| IBIS file stm32h563_573_ufbga169-smps.ibs
[IBIS ver] 4.2
[File name] stm32h563_573_ufbga169-smps.ibs
[File Rev] 1.1
[Date] 07-05-2024
[Source] Data Created at STMicroelectronics
[Notes]  File originated from ELDO simulations.
[Disclaimer]  This information is for modeling purpose only and is
   not guaranteed. The information is subject to change without
   notice.
[Copyright] Copyright 2024 STMicroelectronics Inc.
|   Component stm32h563_573_ufbga169-smps
[Component] stm32h563_573_ufbga169-smps
[Manufacturer] STMicroelectronics
[Package]
| variable   typ   min   max
R_pkg  0  NA  NA
L_pkg  0  NA  NA
C_pkg  0  NA  NA
[Pin]   signal_name   model_name
A1  PI7  io8_ft_i3c_spi
A2  PI6  io8_ft_i3c_spi
A3  VDD  power
A4  VCAP  nc
A5  PB4  io8_ft_i3c_spi
A6  VDDIO2  power
A7  PD5  io8_ft_i3c_spi
A8  VDD  power
A9  PC11  io8_ft_i3c_spi
A10  PC10  io8_ft_i3c_spi
A11  VDD  power
A12  PI3  io8_ft_i3c_spi
A13  PH15  io8_ft_i3c_spi
B1  VDD  power
B2  VSS  gnd
B3  PI5  io8_ft_i3c_spi
B4  VSS  gnd
B5  BOOT0  vpphv
B6  PG15  io8_ft_i3c_spi
B7  PD7  io8_ft_i3c_spi
B8  VSS  gnd
B9  PD1  io8_ft_i3c_spi
B10  PA15  io8_ft_i3c_spi
B11  VSS  gnd
B12  PI0  io8_ft_i3c_spi
B13  PA12  io8usb_ft_i3c_spi_phy
C1  VBAT  power
C2  PE5  io8_ft_i3c_spi
C3  PE2  io8_ft_i3c_spi
C4  PI4  io8_ft_i3c_spi
C5  PE1  io8_ft_i3c_spi
C6  PB6  io8_ft_i3c_spi
C7  PG10  io8_ft_i3c_spi
C8  PD3  io8_ft_i3c_spi
C9  PD0  io8_ft_i3c_spi
C10  PA14  io8_ft_i3c_spi
C11  PI1  io8_ft_i3c_spi
C12  PH13  io8_ft_i3c_spi
C13  PA11  io8usb_ft_i3c_spi_phy
D1  PC14-OSC32_IN  io8_ft_i3c_spi
D2  PE6  io8_ft_i3c_spi
D3  PE4  io8_ft_i3c_spi
D4  PE3  io8_ft_i3c_spi
D5  PE0  io8_ft_i3c_spi
D6  PB7  io8_ft_i3c_spi
D7  PG12  io8_ft_i3c_spi
D8  PD4  io8_ft_i3c_spi
D9  PC12  io8_ft_i3c_spi
D10  PI2  io8_ft_i3c_spi
D11  PH14  io8_ft_i3c_spi
D12  PA13  io8_ft_i3c_spi
D13  VDD  power
E1  PC15-OSC32_OUT  io8_ft_i3c_spi
E2  PF0  io8_ft_i3c_spi
E3  PC13  io8_ft_i3c_spi
E4  PI8  io8_ft_i3c_spi
E5  PB9  io8_ft_i3c_spi
E6  PB5  io8_ft_i3c_spi
E7  PG9  io8_ft_i3c_spi
E8  PD2  io8_ft_i3c_spi
E9  PC8  io8_ft_i3c_spi
E10  PA8  io8_ft_i3c_spi
E11  PA10  io8_ft_i3c_spi
E12  VSS  gnd
E13  VDDUSB  power
F1  PF7  io8_ft_i3c_spi
F2  VSS  gnd
F3  PF1  io8_ft_i3c_spi
F4  PF2  io8_ft_i3c_spi
F5  PB8  io8_ft_i3c_spi
F6  PB3  io8_ft_i3c_spi
F7  PD6  io8_ft_i3c_spi
F8  PG5  io8_ft_i3c_spi
F9  PG7  io8_ft_i3c_spi
F10  PC6  io8_ft_i3c_spi
F11  PC7  io8_ft_i3c_spi
F12  PC9  io8_ft_i3c_spi
F13  PA9  io8_ft_i3c_spi
G1  VDD  power
G2  PF9  io8_ft_i3c_spi
G3  PF5  io8_ft_i3c_spi
G4  PF8  io8_ft_i3c_spi
G5  PF4  io8_ft_i3c_spi
G6  PF3  io8_ft_i3c_spi
G7  PF6  io8_ft_i3c_spi
G8  PD13  io8_ft_i3c_spi
G9  PG3  io8_ft_i3c_spi
G10  PD15  io8_ft_i3c_spi
G11  PG4  io8_ft_i3c_spi
G12  PG6  io8_ft_i3c_spi
G13  PG8  io8_ft_i3c_spi
H1  PH0-OSC_IN  io8_ft_i3c_spi
H2  VSS  gnd
H3  NRST  ioreset_ft_v33
H4  PF10  io8_ft_i3c_spi
H5  PA1  io8_ft_spi_tamp
H6  PB1  io8_ft_spi
H7  PF13  io8_ft_spi
H8  PD11  io8_ft_i3c_spi
H9  PD9  io8_ft_i3c_spi
H10  PB15  io8_ft_spi
H11  PD12  io8_ft_i3c_spi
H12  PD14  io8_ft_i3c_spi
H13  PG2  io8_ft_i3c_spi
J1  PH1  io8_ft_i3c_spi
J2  PC0  io8_ft_spi
J3  PC1  io8_ft_spi
J4  PH2  io8_ft_i3c_spi
J5  PA5  io8_ft_spi
J6  PF11  io8_ft_spi
J7  PF15  io8_ft_i3c_spi
J8  PE8  io8_ft_i3c_spi
J9  PE14  io8_ft_i3c_spi
|J10  PB14  io8usb_ft_pd
J10  PB14 nc
J11  PD8  io8_ft_i3c_spi
J12  VSS  gnd
J13  VDD  power
K1  PC2  io8_ft_spi
K2  PC3  io8_ft_spi
K3  PA0  io8_ft_spi
K4  PA3  io8_ft_spi
K5  PA7  io8_ft_spi
K6  PF12  io8_ft_spi
K7  PG1  io8_ft_i3c_spi
K8  PE13  io8_ft_i3c_spi
K9  PB10  io8_ft_i3c_spi
K10  PH10  io8_ft_i3c_spi
K11  PB12  io8_ft_i3c_spi
|K12  PB13  io8usb_ft_pd
K12  PB13  nc
K13  PD10  io8_ft_i3c_spi
L1  VSSA  nc
L2  VREFM  nc
L3  PA2  io8_ft_spi
L4  PH5  io8_ft_i3c_spi
L5  PC4  io8_ft_spi
L6  PF14  io8_ft_spi
L7  PE7  io8_ft_i3c_spi
L8  PE10  io8_ft_i3c_spi
L9  PE15  io8_ft_i3c_spi
L10  PB11  io8_ft_i3c_spi
L11  PH7  io8_ft_i3c_spi
L12  PH12  io8_ft_i3c_spi
L13  PH11  io8_ft_i3c_spi
M1  VDDA  nc
M2  VREFP  nc
M3  VSS  gnd
M4  PA4  io8_ft_spi
M5  PC5  io8_ft_spi
M6  PG0  io8_ft_i3c_spi
M7  VSS  gnd
M8  PE11  io8_ft_i3c_spi
M9  PE12  io8_ft_i3c_spi
M10  VSSSMPS  nc
M11  VSS  gnd
M12  PH8  io8_ft_i3c_spi
M13  PH9  io8_ft_i3c_spi
N1  PH4  io8_ft_i3c_spi
N2  PH3  io8_ft_i3c_spi
N3  VDD  power
N4  PA6  io8_ft_spi
N5  PB0  io8_ft_spi
N6  PB2  io8_ft_i3c_spi
N7  VDD  power
N8  PE9  io8_ft_i3c_spi
N9  VLXSMPS  nc
N10  VDDSMPS  nc
N11  VCAP  nc
N12  VDD  power
N13  PH6  io8_ft_i3c_spi
[Package Model]   484-ufbga-7x7-169-smps-221014
[Pin Mapping]   pulldown_ref   pullup_ref   | Comment
A1  gndio  vddiom
A2  gndio  vddiom
A3  nc  vddiom
A4  nc  nc
A5  gndio  vddiom  | Depending on IO usage
| A5  gndio  vddmmc  | Depending on IO usage
A6  nc  vddmmc
A7  gndio  vddiom
A8  nc  vddiom
A9  gndio  vddiom
A10  gndio  vddiom
A11  nc  vddiom
A12  gndio  vddiom
A13  gndio  vddiom
B1  nc  vddiom
B2  gndio  nc
B3  gndio  vddiom
B4  gndio  nc
B5  gndio  vddiom  | Depending on IO usage
| B5  gndio  vddmmc  | Depending on IO usage
B6  gndio  vddiom  | Depending on IO usage
| B6  gndio  vddmmc  | Depending on IO usage
B7  gndio  vddiom  | Depending on IO usage
| B7  gndio  vddmmc  | Depending on IO usage
B8  gndio  nc
B9  gndio  vddiom
B10  gndio  vddiom
B11  gndio  nc
B12  gndio  vddiom
B13  gndio  vddiom  | Depending on IO usage
| B13  gndio  vddusb  | Depending on IO usage
C1  nc  vsw
C2  gndio  vddiom
C3  gndio  vddiom
C4  gndio  vddiom
C5  gndio  vddiom  | Depending on IO usage
| C5  gndio  vddmmc  | Depending on IO usage
C6  gndio  vddiom  | Depending on IO usage
| C6  gndio  vddmmc  | Depending on IO usage
C7  gndio  vddiom  | Depending on IO usage
| C7  gndio  vddmmc  | Depending on IO usage
C8  gndio  vddiom
C9  gndio  vddiom
C10  gndio  vddiom
C11  gndio  vddiom
C12  gndio  vddiom
C13  gndio  vddiom  | Depending on IO usage
| C13  gndio  vddusb  | Depending on IO usage
D1  gndio  vddiom  | Depending on IO usage
| D1  gndio  vsw  | Depending on IO usage
D2  gndio  vddiom
D3  gndio  vddiom
D4  gndio  vddiom
D5  gndio  vddiom  | Depending on IO usage
| D5  gndio  vddmmc  | Depending on IO usage
D6  gndio  vddiom  | Depending on IO usage
| D6  gndio  vddmmc  | Depending on IO usage
D7  gndio  vddiom  | Depending on IO usage
| D7  gndio  vddmmc  | Depending on IO usage
D8  gndio  vddiom
D9  gndio  vddiom
D10  gndio  vddiom
D11  gndio  vddiom
D12  gndio  vddiom  | Depending on IO usage
| D12  gndio  vddusb  | Depending on IO usage
D13  nc  vddiom
E1  gndio  vddiom  | Depending on IO usage
| E1  gndio  vsw  | Depending on IO usage
E2  gndio  vddiom
E3  gndio  vddiom  | Depending on IO usage
| E3  gndio  vsw  | Depending on IO usage
E4  gndio  vddiom  | Depending on IO usage
| E4  gndio  vsw  | Depending on IO usage
E5  gndio  vddiom  | Depending on IO usage
| E5  gndio  vddmmc  | Depending on IO usage
E6  gndio  vddiom  | Depending on IO usage
| E6  gndio  vddmmc  | Depending on IO usage
E7  gndio  vddiom  | Depending on IO usage
| E7  gndio  vddmmc  | Depending on IO usage
E8  gndio  vddiom
E9  gndio  vddiom
E10  gndio  vddiom
E11  gndio  vddiom  | Depending on IO usage
| E11  gndio  vddusb  | Depending on IO usage
E12  gndio  nc
E13  nc  vddusb
F1  gndio  vddiom
F2  gndio  nc
F3  gndio  vddiom
F4  gndio  vddiom
F5  gndio  vddiom  | Depending on IO usage
| F5  gndio  vddmmc  | Depending on IO usage
F6  gndio  vddiom  | Depending on IO usage
| F6  gndio  vddmmc  | Depending on IO usage
F7  gndio  vddiom  | Depending on IO usage
| F7  gndio  vddmmc  | Depending on IO usage
F8  gndio  vddiom
F9  gndio  vddiom
F10  gndio  vddiom
F11  gndio  vddiom
F12  gndio  vddiom
F13  gndio  vddiom  | Depending on IO usage
| F13  gndio  vddusb  | Depending on IO usage
G1  nc  vddiom
G2  gndio  vddiom
G3  gndio  vddiom
G4  gndio  vddiom
G5  gndio  vddiom
G6  gndio  vddiom
G7  gndio  vddiom
G8  gndio  vddiom
G9  gndio  vddiom
G10  gndio  vddiom
G11  gndio  vddiom
G12  gndio  vddiom
G13  gndio  vddiom
H1  gndio  vddiom
H2  gndio  nc
H3  gndio  vddiom
H4  gndio  vddiom
H5  gndio  vddiom
H6  gndio  vddiom
H7  gndio  vddiom
H8  gndio  vddiom
H9  gndio  vddiom
H10  gndio  vddiom
H11  gndio  vddiom
H12  gndio  vddiom
H13  gndio  vddiom
J1  gndio  vddiom
J2  gndio  vddiom
J3  gndio  vddiom
J4  gndio  vddiom
J5  gndio  vddiom
J6  gndio  vddiom
J7  gndio  vddiom
J8  gndio  vddiom
J9  gndio  vddiom
|J10  gndio  vddiom
J10  nc nc
J11  gndio  vddiom
J12  gndio  nc
J13  nc  vddiom
K1  gndio  vddiom
K2  gndio  vddiom
K3  gndio  vddiom
K4  gndio  vddiom
K5  gndio  vddiom
K6  gndio  vddiom
K7  gndio  vddiom
K8  gndio  vddiom
K9  gndio  vddiom
K10  gndio  vddiom
K11  gndio  vddiom
|K12  gndio  vddiom
K12  nc nc
K13  gndio  vddiom
L1  nc  nc
L2  nc  nc
L3  gndio  vddiom
L4  gndio  vddiom
L5  gndio  vddiom
L6  gndio  vddiom
L7  gndio  vddiom
L8  gndio  vddiom
L9  gndio  vddiom
L10  gndio  vddiom
L11  gndio  vddiom
L12  gndio  vddiom
L13  gndio  vddiom
M1  nc  nc
M2  nc  nc
M3  gndio  nc
M4  gndio  vddiom
M5  gndio  vddiom
M6  gndio  vddiom
M7  gndio  nc
M8  gndio  vddiom
M9  gndio  vddiom
M10  nc  nc
M11  gndio  nc
M12  gndio  vddiom
M13  gndio  vddiom
N1  gndio  vddiom
N2  gndio  vddiom
N3  nc  vddiom
N4  gndio  vddiom
N5  gndio  vddiom
N6  gndio  vddiom
N7  nc  vddiom
N8  gndio  vddiom
N9  nc  nc
N10  nc  nc
N11  nc  nc
N12  nc  vddiom
N13  gndio  vddiom
[Model Selector] io8_ft_i3c_spi
io8_ft_spi_ls_1v2 "io8_ft spi low speed @ 1.2V"
io8_ft_spi_ls_1v8 "io8_ft spi low speed @ 1.8V"
io8_ft_spi_ls_3v3 "io8_ft spi low speed @ 3.3V"
io8_ft_spi_ms_1v2 "io8_ft spi med speed @ 1.2V"
io8_ft_spi_ms_1v8 "io8_ft spi med speed @ 1.8V"
io8_ft_spi_ms_3v3 "io8_ft spi med speed @ 3.3V"
io8_ft_spi_fs_1v2 "io8_ft spi fast speed @ 1.2V"
io8_ft_spi_fs_1v8 "io8_ft spi fast speed @ 1.8V"
io8_ft_spi_fs_3v3 "io8_ft spi fast speed @ 3.3V"
io8_ft_spi_hs_1v2 "io8_ft spi high speed @ 1.2V"
io8_ft_spi_hs_1v8 "io8_ft spi high speed @ 1.8V"
io8_ft_spi_hs_3v3 "io8_ft spi high speed @ 3.3V"
io8_ft_hslv_spi_ls_1v2 "io8_ft spi hslv low speed @ 1.2V"
io8_ft_hslv_spi_ls_1v8 "io8_ft spi hslv low speed @ 1.8V"
io8_ft_hslv_spi_ls_2v5 "io8_ft spi hslv low speed @ 2.5V"
io8_ft_hslv_spi_ms_1v2 "io8_ft spi hslv med speed @ 1.2V"
io8_ft_hslv_spi_ms_1v8 "io8_ft spi hslv med speed @ 1.8V"
io8_ft_hslv_spi_ms_2v5 "io8_ft spi hslv med speed @ 2.5V"
io8_ft_hslv_spi_fs_1v2 "io8_ft spi hslv fast speed @ 1.2V"
io8_ft_hslv_spi_fs_1v8 "io8_ft spi hslv fast speed @ 1.8V"
io8_ft_hslv_spi_fs_2v5 "io8_ft spi hslv fast speed @ 2.5V"
io8_ft_hslv_spi_hs_1v2 "io8_ft spi hslv high speed @ 1.2V"
io8_ft_hslv_spi_hs_1v8 "io8_ft spi hslv high speed @ 1.8V"
io8_ft_hslv_spi_hs_2v5 "io8_ft spi hslv high speed @ 2.5V"
io8_ft_i3c_spi_ls_1v2 "io8_ft i3c spi open-drain low speed @ 1.2V"
io8_ft_i3c_spi_ls_1v8 "io8_ft i3c spi open-drain low speed @ 1.8V"
io8_ft_i3c_spi_ls_3v3 "io8_ft i3c spi open-drain low speed @ 3.3V"
io8_ft_i3c_spi_ms_1v2 "io8_ft i3c spi open-drain med speed @ 1.2V"
io8_ft_i3c_spi_ms_1v8 "io8_ft i3c spi open-drain med speed @ 1.8V"
io8_ft_i3c_spi_ms_3v3 "io8_ft i3c spi open-drain med speed @ 3.3V"
io8_ft_i3c_spi_fs_1v2 "io8_ft i3c spi open-drain fast speed @ 1.2V"
io8_ft_i3c_spi_fs_1v8 "io8_ft i3c spi open-drain fast speed @ 1.8V"
io8_ft_i3c_spi_fs_3v3 "io8_ft i3c spi open-drain fast speed @ 3.3V"
io8_ft_i3c_spi_hs_1v2 "io8_ft i3c spi open-drain high speed @ 1.2V"
io8_ft_i3c_spi_hs_1v8 "io8_ft i3c spi open-drain high speed @ 1.8V"
io8_ft_i3c_spi_hs_3v3 "io8_ft i3c spi open-drain high speed @ 3.3V"
io8_ft_hslv_i3c_spi_ls_1v2 "io8_ft hslv i3c spi open-drain low speed @ 1.2V"
io8_ft_hslv_i3c_spi_ls_1v8 "io8_ft hslv i3c spi open-drain low speed @ 1.8V"
io8_ft_hslv_i3c_spi_ls_2v5 "io8_ft hslv i3c spi open-drain low speed @ 2.5V"
io8_ft_hslv_i3c_spi_ms_1v2 "io8_ft hslv i3c spi open-drain med speed @ 1.2V"
io8_ft_hslv_i3c_spi_ms_1v8 "io8_ft hslv i3c spi open-drain med speed @ 1.8V"
io8_ft_hslv_i3c_spi_ms_2v5 "io8_ft hslv i3c spi open-drain med speed @ 2.5V"
io8_ft_hslv_i3c_spi_fs_1v2 "io8_ft hslv i3c spi open-drain fast speed @ 1.2V"
io8_ft_hslv_i3c_spi_fs_1v8 "io8_ft hslv i3c spi open-drain fast speed @ 1.8V"
io8_ft_hslv_i3c_spi_fs_2v5 "io8_ft hslv i3c spi open-drain fast speed @ 2.5V"
io8_ft_hslv_i3c_spi_hs_1v2 "io8_ft hslv i3c spi open-drain high speed @ 1.2V"
io8_ft_hslv_i3c_spi_hs_1v8 "io8_ft hslv i3c spi open-drain high speed @ 1.8V"
io8_ft_hslv_i3c_spi_hs_2v5 "io8_ft hslv i3c spi open-drain high speed @ 2.5V"
io8_ft_i3c_fmp_spi_3v3 "io8_ft i3c fm+ spi open-drain @ 3.3V"
io8_ft_i3c_fmp_spi_1v8 "io8_ft i3c fm+ spi open-drain @ 1.8V"
io8_ft_i3c_fmp_spi_1v2 "io8_ft i3c fm+ spi open-drain @ 1.2V"
[Model Selector] io8_ft_spi
io8_ft_spi_ls_1v2 "io8_ft spi low speed @ 1.2V"
io8_ft_spi_ls_1v8 "io8_ft spi low speed @ 1.8V"
io8_ft_spi_ls_3v3 "io8_ft spi low speed @ 3.3V"
io8_ft_spi_ms_1v2 "io8_ft spi med speed @ 1.2V"
io8_ft_spi_ms_1v8 "io8_ft spi med speed @ 1.8V"
io8_ft_spi_ms_3v3 "io8_ft spi med speed @ 3.3V"
io8_ft_spi_fs_1v2 "io8_ft spi fast speed @ 1.2V"
io8_ft_spi_fs_1v8 "io8_ft spi fast speed @ 1.8V"
io8_ft_spi_fs_3v3 "io8_ft spi fast speed @ 3.3V"
io8_ft_spi_hs_1v2 "io8_ft spi high speed @ 1.2V"
io8_ft_spi_hs_1v8 "io8_ft spi high speed @ 1.8V"
io8_ft_spi_hs_3v3 "io8_ft spi high speed @ 3.3V"
io8_ft_hslv_spi_ls_1v2 "io8_ft spi hslv low speed @ 1.2V"
io8_ft_hslv_spi_ls_1v8 "io8_ft spi hslv low speed @ 1.8V"
io8_ft_hslv_spi_ls_2v5 "io8_ft spi hslv low speed @ 2.5V"
io8_ft_hslv_spi_ms_1v2 "io8_ft spi hslv med speed @ 1.2V"
io8_ft_hslv_spi_ms_1v8 "io8_ft spi hslv med speed @ 1.8V"
io8_ft_hslv_spi_ms_2v5 "io8_ft spi hslv med speed @ 2.5V"
io8_ft_hslv_spi_fs_1v2 "io8_ft spi hslv fast speed @ 1.2V"
io8_ft_hslv_spi_fs_1v8 "io8_ft spi hslv fast speed @ 1.8V"
io8_ft_hslv_spi_fs_2v5 "io8_ft spi hslv fast speed @ 2.5V"
io8_ft_hslv_spi_hs_1v2 "io8_ft spi hslv high speed @ 1.2V"
io8_ft_hslv_spi_hs_1v8 "io8_ft spi hslv high speed @ 1.8V"
io8_ft_hslv_spi_hs_2v5 "io8_ft spi hslv high speed @ 2.5V"
[Model Selector] io8_ft_spi_tamp
io8_ft_spi_ls_1v2 "io8_ft spi low speed @ 1.2V"
io8_ft_spi_ls_1v8 "io8_ft spi low speed @ 1.8V"
io8_ft_spi_ls_3v3 "io8_ft spi low speed @ 3.3V"
io8_ft_spi_ms_1v2 "io8_ft spi med speed @ 1.2V"
io8_ft_spi_ms_1v8 "io8_ft spi med speed @ 1.8V"
io8_ft_spi_ms_3v3 "io8_ft spi med speed @ 3.3V"
io8_ft_spi_fs_1v2 "io8_ft spi fast speed @ 1.2V"
io8_ft_spi_fs_1v8 "io8_ft spi fast speed @ 1.8V"
io8_ft_spi_fs_3v3 "io8_ft spi fast speed @ 3.3V"
io8_ft_spi_hs_1v2 "io8_ft spi high speed @ 1.2V"
io8_ft_spi_hs_1v8 "io8_ft spi high speed @ 1.8V"
io8_ft_spi_hs_3v3 "io8_ft spi high speed @ 3.3V"
io8_ft_hslv_spi_ls_1v2 "io8_ft spi hslv low speed @ 1.2V"
io8_ft_hslv_spi_ls_1v8 "io8_ft spi hslv low speed @ 1.8V"
io8_ft_hslv_spi_ls_2v5 "io8_ft spi hslv low speed @ 2.5V"
io8_ft_hslv_spi_ms_1v2 "io8_ft spi hslv med speed @ 1.2V"
io8_ft_hslv_spi_ms_1v8 "io8_ft spi hslv med speed @ 1.8V"
io8_ft_hslv_spi_ms_2v5 "io8_ft spi hslv med speed @ 2.5V"
io8_ft_hslv_spi_fs_1v2 "io8_ft spi hslv fast speed @ 1.2V"
io8_ft_hslv_spi_fs_1v8 "io8_ft spi hslv fast speed @ 1.8V"
io8_ft_hslv_spi_fs_2v5 "io8_ft spi hslv fast speed @ 2.5V"
io8_ft_hslv_spi_hs_1v2 "io8_ft spi hslv high speed @ 1.2V"
io8_ft_hslv_spi_hs_1v8 "io8_ft spi hslv high speed @ 1.8V"
io8_ft_hslv_spi_hs_2v5 "io8_ft spi hslv high speed @ 2.5V"
io8_ft_tamp_v33_1v2 "io8_ft tamp V33 @ 1.2V"
io8_ft_tamp_v33_1v8 "io8_ft tamp V33 @ 1.2V"
io8_ft_tamp_v33_3v3 "io8_ft tamp V33 @ 1.2V"
[Model Selector] io8usb_ft_i3c_spi_phy
io8_ft_spi_ls_1v2 "io8_ft spi low speed @ 1.2V"
io8_ft_spi_ls_1v8 "io8_ft spi low speed @ 1.8V"
io8_ft_spi_ls_3v3 "io8_ft spi low speed @ 3.3V"
io8_ft_spi_ms_1v2 "io8_ft spi med speed @ 1.2V"
io8_ft_spi_ms_1v8 "io8_ft spi med speed @ 1.8V"
io8_ft_spi_ms_3v3 "io8_ft spi med speed @ 3.3V"
io8_ft_spi_fs_1v2 "io8_ft spi fast speed @ 1.2V"
io8_ft_spi_fs_1v8 "io8_ft spi fast speed @ 1.8V"
io8_ft_spi_fs_3v3 "io8_ft spi fast speed @ 3.3V"
io8_ft_spi_hs_1v2 "io8_ft spi high speed @ 1.2V"
io8_ft_spi_hs_1v8 "io8_ft spi high speed @ 1.8V"
io8_ft_spi_hs_3v3 "io8_ft spi high speed @ 3.3V"
io8_ft_hslv_spi_ls_1v2 "io8_ft spi hslv low speed @ 1.2V"
io8_ft_hslv_spi_ls_1v8 "io8_ft spi hslv low speed @ 1.8V"
io8_ft_hslv_spi_ls_2v5 "io8_ft spi hslv low speed @ 2.5V"
io8_ft_hslv_spi_ms_1v2 "io8_ft spi hslv med speed @ 1.2V"
io8_ft_hslv_spi_ms_1v8 "io8_ft spi hslv med speed @ 1.8V"
io8_ft_hslv_spi_ms_2v5 "io8_ft spi hslv med speed @ 2.5V"
io8_ft_hslv_spi_fs_1v2 "io8_ft spi hslv fast speed @ 1.2V"
io8_ft_hslv_spi_fs_1v8 "io8_ft spi hslv fast speed @ 1.8V"
io8_ft_hslv_spi_fs_2v5 "io8_ft spi hslv fast speed @ 2.5V"
io8_ft_hslv_spi_hs_1v2 "io8_ft spi hslv high speed @ 1.2V"
io8_ft_hslv_spi_hs_1v8 "io8_ft spi hslv high speed @ 1.8V"
io8_ft_hslv_spi_hs_2v5 "io8_ft spi hslv high speed @ 2.5V"
io8_ft_i3c_spi_ls_1v2 "io8_ft i3c spi open-drain low speed @ 1.2V"
io8_ft_i3c_spi_ls_1v8 "io8_ft i3c spi open-drain low speed @ 1.8V"
io8_ft_i3c_spi_ls_3v3 "io8_ft i3c spi open-drain low speed @ 3.3V"
io8_ft_i3c_spi_ms_1v2 "io8_ft i3c spi open-drain med speed @ 1.2V"
io8_ft_i3c_spi_ms_1v8 "io8_ft i3c spi open-drain med speed @ 1.8V"
io8_ft_i3c_spi_ms_3v3 "io8_ft i3c spi open-drain med speed @ 3.3V"
io8_ft_i3c_spi_fs_1v2 "io8_ft i3c spi open-drain fast speed @ 1.2V"
io8_ft_i3c_spi_fs_1v8 "io8_ft i3c spi open-drain fast speed @ 1.8V"
io8_ft_i3c_spi_fs_3v3 "io8_ft i3c spi open-drain fast speed @ 3.3V"
io8_ft_i3c_spi_hs_1v2 "io8_ft i3c spi open-drain high speed @ 1.2V"
io8_ft_i3c_spi_hs_1v8 "io8_ft i3c spi open-drain high speed @ 1.8V"
io8_ft_i3c_spi_hs_3v3 "io8_ft i3c spi open-drain high speed @ 3.3V"
io8_ft_hslv_i3c_spi_ls_1v2 "io8_ft hslv i3c spi open-drain low speed @ 1.2V"
io8_ft_hslv_i3c_spi_ls_1v8 "io8_ft hslv i3c spi open-drain low speed @ 1.8V"
io8_ft_hslv_i3c_spi_ls_2v5 "io8_ft hslv i3c spi open-drain low speed @ 2.5V"
io8_ft_hslv_i3c_spi_ms_1v2 "io8_ft hslv i3c spi open-drain med speed @ 1.2V"
io8_ft_hslv_i3c_spi_ms_1v8 "io8_ft hslv i3c spi open-drain med speed @ 1.8V"
io8_ft_hslv_i3c_spi_ms_2v5 "io8_ft hslv i3c spi open-drain med speed @ 2.5V"
io8_ft_hslv_i3c_spi_fs_1v2 "io8_ft hslv i3c spi open-drain fast speed @ 1.2V"
io8_ft_hslv_i3c_spi_fs_1v8 "io8_ft hslv i3c spi open-drain fast speed @ 1.8V"
io8_ft_hslv_i3c_spi_fs_2v5 "io8_ft hslv i3c spi open-drain fast speed @ 2.5V"
io8_ft_hslv_i3c_spi_hs_1v2 "io8_ft hslv i3c spi open-drain high speed @ 1.2V"
io8_ft_hslv_i3c_spi_hs_1v8 "io8_ft hslv i3c spi open-drain high speed @ 1.8V"
io8_ft_hslv_i3c_spi_hs_2v5 "io8_ft hslv i3c spi open-drain high speed @ 2.5V"
io8_ft_i3c_fmp_spi_3v3 "io8_ft i3c fm+ spi open-drain @ 3.3V"
io8_ft_i3c_fmp_spi_1v8 "io8_ft i3c fm+ spi open-drain @ 1.8V"
io8_ft_i3c_fmp_spi_1v2 "io8_ft i3c fm+ spi open-drain @ 1.2V"
io8usb_ft_phy_ls_2v5 "iousb ft low speed @ 2.5V"
io8usb_ft_phy_ls_3v3 "iousb ft low speed @ 3.3V"
io8usb_ft_phy_fs_2v5 "iousb ft fast speed @ 2.5V"
io8usb_ft_phy_fs_3v3 "iousb ft fast speed @ 3.3V"
[Model Selector] ioreset_ft_v33
ioreset_ft_v33_1v2 "Reset PAD. 5V tolerant. 1.2V range"
ioreset_ft_v33_1v8 "Reset PAD. 5V tolerant. 1.8V range"
ioreset_ft_v33_3v3 "Reset PAD. 5V tolerant. 3.3V range"
[Model Selector] vpphv
vpphv_1v2 "Flash Test cell v33 = 1.2 V range"
vpphv_1v8 "Flash Test cell v33 = 1.8 V range"
vpphv_3v3 "Flash Test cell v33 = 3.3 V range"
[Define Package Model]  484-ufbga-7x7-169-smps-221014
[Manufacturer]  unknown
[OEM]  unknown
[Description]  unknown
[Number Of Pins]  150
[Pin Numbers]
| Pin Name Terminal   Net Name   Starting Node   Ending Node
B5 | BOOT0
H3 | NRST
K3 | PA0
H5 | PA1
L3 | PA2
K4 | PA3
M4 | PA4
J5 | PA5
N4 | PA6
K5 | PA7
E10 | PA8
F13 | PA9
E11 | PA10
C13 | PA11
B13 | PA12
D12 | PA13
C10 | PA14
B10 | PA15
N5 | PB0
H6 | PB1
N6 | PB2
F6 | PB3
A5 | PB4
E6 | PB5
C6 | PB6
D6 | PB7
F5 | PB8
E5 | PB9
K9 | PB10
L10 | PB11
K11 | PB12
K12 | PB13
J10 | PB14
H10 | PB15
J2 | PC0
J3 | PC1
K1 | PC2
K2 | PC3
L5 | PC4
M5 | PC5
F10 | PC6
F11 | PC7
E9 | PC8
F12 | PC9
A10 | PC10
A9 | PC11
D9 | PC12
E3 | PC13
D1 | PC14-OSC32_IN
E1 | PC15-OSC32_OUT
C9 | PD0
B9 | PD1
E8 | PD2
C8 | PD3
D8 | PD4
A7 | PD5
F7 | PD6
B7 | PD7
J11 | PD8
H9 | PD9
K13 | PD10
H8 | PD11
H11 | PD12
G8 | PD13
H12 | PD14
G10 | PD15
D5 | PE0
C5 | PE1
C3 | PE2
D4 | PE3
D3 | PE4
C2 | PE5
D2 | PE6
L7 | PE7
J8 | PE8
N8 | PE9
L8 | PE10
M8 | PE11
M9 | PE12
K8 | PE13
J9 | PE14
L9 | PE15
E2 | PF0
F3 | PF1
F4 | PF2
G6 | PF3
G5 | PF4
G3 | PF5
G7 | PF6
F1 | PF7
G4 | PF8
G2 | PF9
H4 | PF10
J6 | PF11
K6 | PF12
H7 | PF13
L6 | PF14
J7 | PF15
M6 | PG0
K7 | PG1
H13 | PG2
G9 | PG3
G11 | PG4
F8 | PG5
G12 | PG6
F9 | PG7
G13 | PG8
E7 | PG9
C7 | PG10
D7 | PG12
B6 | PG15
H1 | PH0-OSC_IN
J1 | PH1-OSC_OUT
J4 | PH2
N2 | PH3
N1 | PH4
L4 | PH5
N13 | PH6
L11 | PH7
M12 | PH8
M13 | PH9
K10 | PH10
L13 | PH11
L12 | PH12
C12 | PH13
D11 | PH14
A13 | PH15
B12 | PI0
C11 | PI1
D10 | PI2
A12 | PI3
C4 | PI4
B3 | PI5
A2 | PI6
A1 | PI7
E4 | PI8
C1 | VBAT
N11 | VCAP
A4 | VCAP
E13 | VDDUSB
A3 | VDD
M1 | VDDA
N10 | VDDSMPS
A6 | VDDIO2
N9 | VLXSMPS
L2 | VREFM
M2 | VREFP
B2 | VSS
L1 | VSSA
M10 | VSSSMPS
|[Merged Pins]  A3
|A8  |  VDD
|A11  |  VDD
|B1  |  VDD
|D13  |  VDD
|G1  |  VDD
|J13  |  VDD
|N3  |  VDD
|N7  |  VDD
|N12  |  VDD
|[Merged Pins]  B2
|B4  |  VSS
|B8  |  VSS
|B11  |  VSS
|E12  |  VSS
|F2  |  VSS
|H2  |  VSS
|J12  |  VSS
|M3  |  VSS
|M7  |  VSS
|M11  |  VSS
[Model Data]
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[End Model Data]
[End Package Model]
|End [Component]
| Models and submodels in the file (64): io8_ft_hslv_i3c_spi_fs_1v2 (I/O_open_drain), io8_ft_hslv_i3c_spi_fs_1v8 (I/O_open_drain), io8_ft_hslv_i3c_spi_fs_2v5 (I/O_open_drain), io8_ft_hslv_i3c_spi_hs_1v2 (I/O_open_drain), io8_ft_hslv_i3c_spi_hs_1v8 (I/O_open_drain), io8_ft_hslv_i3c_spi_hs_2v5 (I/O_open_drain), io8_ft_hslv_i3c_spi_ls_1v2 (I/O_open_drain), io8_ft_hslv_i3c_spi_ls_1v8 (I/O_open_drain), io8_ft_hslv_i3c_spi_ls_2v5 (I/O_open_drain), io8_ft_hslv_i3c_spi_ms_1v2 (I/O_open_drain), io8_ft_hslv_i3c_spi_ms_1v8 (I/O_open_drain), io8_ft_hslv_i3c_spi_ms_2v5 (I/O_open_drain), io8_ft_hslv_spi_fs_1v2 (I/O), io8_ft_hslv_spi_fs_1v8 (I/O), io8_ft_hslv_spi_fs_2v5 (I/O), io8_ft_hslv_spi_hs_1v2 (I/O), io8_ft_hslv_spi_hs_1v8 (I/O), io8_ft_hslv_spi_hs_2v5 (I/O), io8_ft_hslv_spi_ls_1v2 (I/O), io8_ft_hslv_spi_ls_1v8 (I/O), io8_ft_hslv_spi_ls_2v5 (I/O), io8_ft_hslv_spi_ms_1v2 (I/O), io8_ft_hslv_spi_ms_1v8 (I/O), io8_ft_hslv_spi_ms_2v5 (I/O), io8_ft_i3c_fmp_spi_1v2 (I/O_open_drain), io8_ft_i3c_fmp_spi_1v8 (I/O_open_drain), io8_ft_i3c_fmp_spi_3v3 (I/O_open_drain), io8_ft_i3c_spi_fs_1v2 (I/O_open_drain), io8_ft_i3c_spi_fs_1v8 (I/O_open_drain), io8_ft_i3c_spi_fs_3v3 (I/O_open_drain), io8_ft_i3c_spi_hs_1v2 (I/O_open_drain), io8_ft_i3c_spi_hs_1v8 (I/O_open_drain), io8_ft_i3c_spi_hs_3v3 (I/O_open_drain), io8_ft_i3c_spi_ls_1v2 (I/O_open_drain), io8_ft_i3c_spi_ls_1v8 (I/O_open_drain), io8_ft_i3c_spi_ls_3v3 (I/O_open_drain), io8_ft_i3c_spi_ms_1v2 (I/O_open_drain), io8_ft_i3c_spi_ms_1v8 (I/O_open_drain), io8_ft_i3c_spi_ms_3v3 (I/O_open_drain), io8_ft_spi_fs_1v2 (I/O), io8_ft_spi_fs_1v8 (I/O), io8_ft_spi_fs_3v3 (I/O), io8_ft_spi_hs_1v2 (I/O), io8_ft_spi_hs_1v8 (I/O), io8_ft_spi_hs_3v3 (I/O), io8_ft_spi_ls_1v2 (I/O), io8_ft_spi_ls_1v8 (I/O), io8_ft_spi_ls_3v3 (I/O), io8_ft_spi_ms_1v2 (I/O), io8_ft_spi_ms_1v8 (I/O), io8_ft_spi_ms_3v3 (I/O), io8_ft_tamp_v33_1v2 (I/O), io8_ft_tamp_v33_1v8 (I/O), io8_ft_tamp_v33_3v3 (I/O), io8usb_ft_phy_fs_2v5 (I/O), io8usb_ft_phy_fs_3v3 (I/O), io8usb_ft_phy_ls_2v5 (I/O), io8usb_ft_phy_ls_3v3 (I/O), ioreset_ft_v33_1v2 (I/O_open_drain), ioreset_ft_v33_1v8 (I/O_open_drain), ioreset_ft_v33_3v3 (I/O_open_drain), vpphv_1v2 (Input), vpphv_1v8 (Input), vpphv_3v3 (Input)
